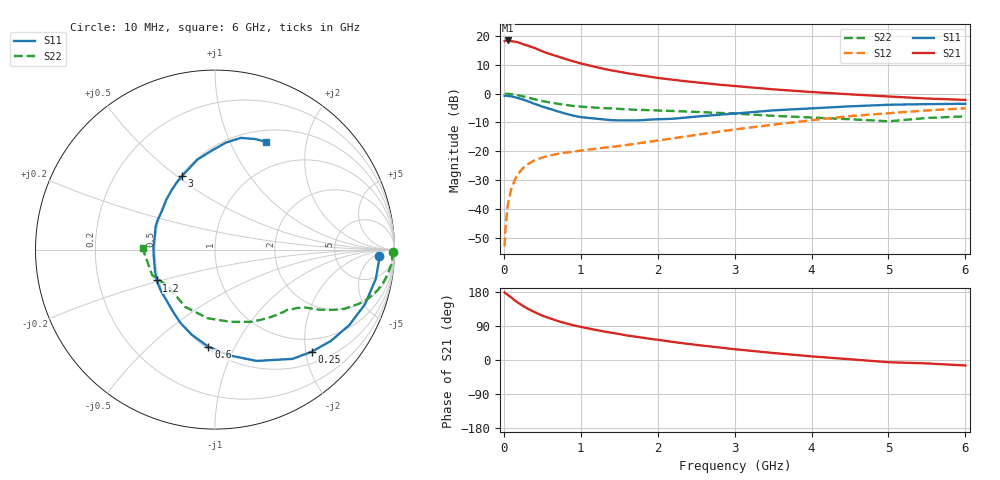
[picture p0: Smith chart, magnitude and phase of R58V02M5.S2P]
! SIEMENS Small Signal Semiconductors
! BFR183
! Si NPN RF Bipolar Junction Transistor in SOT23
! VCE = 8 V  IC = 2.5 mA
! Common Emitter S-Parameters:  May  1996
# GHz  S  MA  R  50
!  f  S11  S21  S12  S22
! GHz  MAG  ANG  MAG  ANG  MAG  ANG  MAG  ANG
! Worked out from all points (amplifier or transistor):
!   36 points, 10 MHz to 6 GHz, reference 50 ohm
!   highest |S21| = 18.3 dB at 50 MHz (marker M1)
!   |S21| within 3 dB of that: start of sweep to 434 MHz
!   unconditionally stable (mu >= 1): 1.354 GHz to 2.836 GHz
!   at 250 MHz: K = 0.27, MSG = 21.4 dB, |S12| = -25.7 dB
!   at 1.4 GHz: K = 1.02, MAG = 12.3 dB, |S12| = -18.5 dB
!   at 6 GHz: K = 0.88, MSG = 1.4 dB, |S12| = -5.1 dB
!   S11 on the Smith chart (normalised r, x): 10 MHz: 19, -8; 250 MHz: 0.72, -2.12; 600 MHz: 0.52, -0.79; 1.2 GHz: 0.49, -0.19; 3 GHz: 0.51, +0.52; 6 GHz: 0.64, +1.38
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0.01  0.9142 -2.1  8.071 178.6  0.0023 86.0  0.9933 -0.8
0.02  0.9153 -4.1  8.177 176.6  0.0046 91.7  0.9868 -1.6
0.05  0.9107 -10.3  8.256 172.0  0.0117 85.1  0.9898 -4.2
0.15  0.8584 -29.3  7.857 156.0  0.0339 74.0  0.951 -12.0
0.2  0.8223 -38.2  7.547 149.2  0.0429 69.4  0.9222 -15.3
0.25  0.7839 -46.5  7.117 142.7  0.0517 64.8  0.8905 -18.2
0.3  0.7468 -54.6  6.784 136.4  0.0588 62.2  0.859 -20.5
0.4  0.6623 -69.5  6.113 126.3  0.0701 56.2  0.7948 -24.5
0.5  0.5945 -82.3  5.358 117.1  0.0782 52.3  0.7393 -27.0
0.6  0.5423 -93.9  4.804 109.8  0.0853 49.9  0.7002 -28.7
0.7  0.4917 -105.3  4.374 103.0  0.0905 47.9  0.6664 -30.1
0.8  0.4506 -115.5  3.954 97.1  0.0949 46.7  0.6363 -31.2
0.9  0.4152 -124.8  3.613 91.9  0.0993 46.8  0.611 -32.1
1.1  0.3787 -143.0  3.075 83.2  0.107 47.2  0.5804 -33.9
1.2  0.3671 -152.1  2.862 79.1  0.1109 47.4  0.5688 -34.8
1.6  0.3432 177.7  2.247 64.8  0.1294 50.4  0.5339 -38.9
2.2  0.3662 143.9  1.726 47.6  0.1683 54.3  0.4984 -47.2
3  0.4497 113.9  1.349 28.5  0.2391 53.2  0.4497 -63.5
3.5  0.5109 101.1  1.181 18.5  0.2888 49.4  0.412 -77.8
4.5  0.6001 84.0  0.968 2.0  0.4066 38.6  0.3595 -117.7
5.5  0.6551 70.1  0.819 -9.0  0.5094 25.0  0.3778 -158.0
6  0.6646 64.7  0.775 -14.5  0.556 16.2  0.4034 179.0
